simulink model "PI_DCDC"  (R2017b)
settings: Solver=FixedStepDiscrete  StartTime=0.0  StopTime=0.02  FixedStep=2e-5  RelTol=1e-3  EnableMultiTasking=on
libraries: SCIDEAM_BLOCKS_100 x2

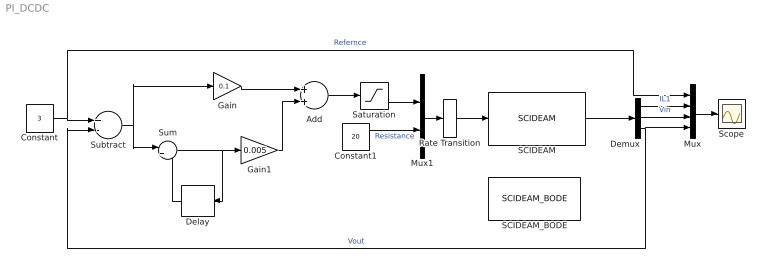
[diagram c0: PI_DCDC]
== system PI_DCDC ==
  Add : Sum
  Constant : Constant  Value=3
  Constant1 : Constant  Value=20
  Delay : Delay  DelayLength=1  InitialCondition=0
  Demux : Demux  Outputs=3
  Gain : Gain  Gain=0.1
  Gain1 : Gain  Gain=0.005
  Mux : Mux
  Mux1 : Mux  Inputs=2
  Rate Transition : RateTransition  OutPortSampleTime=2e-5
  SCIDEAM : SCIDEAM_BLOCKS_100/SCIDEAM  ScalCliPath=Scal.Cli.exe  CvtFilePath=BuckConverter.cvt2  SimulationMode=Waveform  WaveformStartTime=0.019  FrequencyResponseAnalysisStartTime=0.04  VasSymbols=<empty>  FromSignatures=<empty>  ToSignatures=<empty>  PhaseFold=on  InputWidth=2  OutputWidth=3
  SCIDEAM_BODE : SCIDEAM_BLOCKS_100/SCIDEAM_BODE  EnabledAutoBode=on
  Saturation : Saturate  UpperLimit=1  LowerLimit=0
  Scope : Scope
  Subtract : Sum  Inputs=+-
  Sum : Sum  Inputs=|++
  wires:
  Constant/1 -> Mux/1, Subtract/1  "Refernce"
  Subtract/1 -> Gain/1, Sum/1
  Gain/1 -> Add/1
  Add/1 -> Saturation/1
  Gain1/1 -> Add/2
  Sum/1 -> Delay/1, Gain1/1
  Delay/1 -> Sum/2
  Mux/1 -> Scope/1
  Demux/1 -> Mux/2  "IL1"
  Demux/2 -> Mux/3  "Vin"
  SCIDEAM/1 -> Demux/1
  Rate Transition/1 -> SCIDEAM/1
  Demux/3 -> Subtract/2, Mux/4  "Vout"
  Mux1/1 -> Rate Transition/1
  Saturation/1 -> Mux1/1
  Constant1/1 -> Mux1/2  "Resistance"
